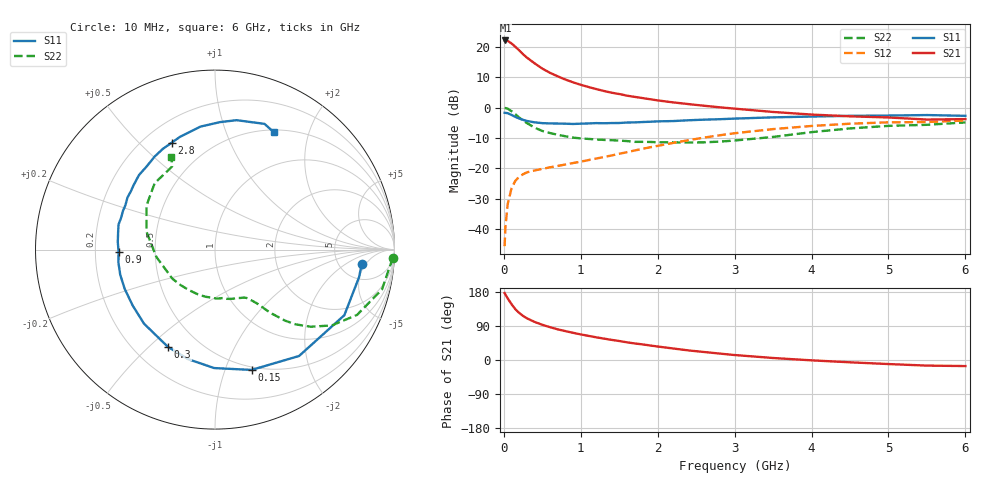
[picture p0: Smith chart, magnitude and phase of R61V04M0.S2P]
! SIEMENS Small Signal Semiconductors
! BFR193
! Si NPN RF Bipolar Junction Transistor in SOT23
! VCE = 1 V  IC = 4 mA
! Common Emitter S-Parameters:  May  1996
# GHz  S  MA  R  50
!  f  S11  S21  S12  S22
! GHz  MAG  ANG  MAG  ANG  MAG  ANG  MAG  ANG
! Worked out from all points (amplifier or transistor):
!   36 points, 10 MHz to 6 GHz, reference 50 ohm
!   highest |S21| = 22.0 dB at 20 MHz (marker M1)
!   |S21| within 3 dB of that: start of sweep to 189.3 MHz
!   unconditionally stable (mu >= 1): 927 MHz to 2.194 GHz
!   at 250 MHz: K = 0.37, MSG = 19.7 dB, |S12| = -21.9 dB
!   at 1.4 GHz: K = 1.09, MAG = 8.4 dB, |S12| = -15.7 dB
!   at 6 GHz: K = 0.99, MSG = 0.2 dB, |S12| = -4.3 dB
!   S11 on the Smith chart (normalised r, x): 10 MHz: 8.26, -4.01; 150 MHz: 0.47, -1.24; 300 MHz: 0.34, -0.57; 900 MHz: 0.30, -0.01; 2.8 GHz: 0.31, +0.63; 6 GHz: 0.53, +1.49
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0.01  0.8218 -5.5  12.61 176.7  0.0053 84.9  0.9914 -2.7
0.02  0.8171 -10.9  12.62 172.9  0.0108 84.3  0.9791 -5.4
0.05  0.808 -26.9  12.45 162.5  0.026 76.7  0.9566 -13.4
0.1  0.7554 -51.7  11.27 147.3  0.0473 64.8  0.871 -24.7
0.15  0.7006 -73.1  9.934 133.9  0.0628 55.8  0.7757 -33.0
0.2  0.66 -90.4  8.682 124.1  0.0733 50.1  0.6844 -38.9
0.25  0.6284 -103.9  7.486 116.3  0.0804 45.9  0.6112 -42.9
0.3  0.6022 -115.8  6.603 110.0  0.0863 43.8  0.5561 -45.4
0.4  0.5715 -133.8  5.317 100.5  0.0927 41.3  0.4678 -48.8
0.5  0.5545 -145.8  4.357 92.9  0.0984 40.7  0.4125 -50.7
0.6  0.5487 -156.5  3.714 86.6  0.1044 41.0  0.3813 -52.0
0.7  0.5463 -165.2  3.252 80.9  0.11 42.2  0.357 -53.6
0.9  0.5372 -178.5  2.593 71.7  0.1228 45.8  0.3207 -57.0
1.1  0.5482 170.0  2.173 63.7  0.1372 48.7  0.3055 -61.8
1.3  0.5523 161.3  1.872 56.5  0.1542 51.1  0.2943 -66.9
1.6  0.5674 149.3  1.566 46.7  0.1851 53.3  0.2816 -76.9
2.2  0.5997 129.4  1.215 30.4  0.2625 52.4  0.2681 -101.8
2.8  0.6428 112.0  1.01 17.1  0.3498 46.1  0.2756 -134.3
3.5  0.6902 96.7  0.846 5.3  0.4426 34.8  0.3291 -172.8
4.5  0.7311 80.5  0.717 -6.1  0.5427 17.8  0.4538 147.2
5.5  0.7529 68.5  0.635 -14.8  0.5784 1.5  0.5208 117.3
6  0.731 63.3  0.646 -16.0  0.612 -3.2  0.57 115.2
